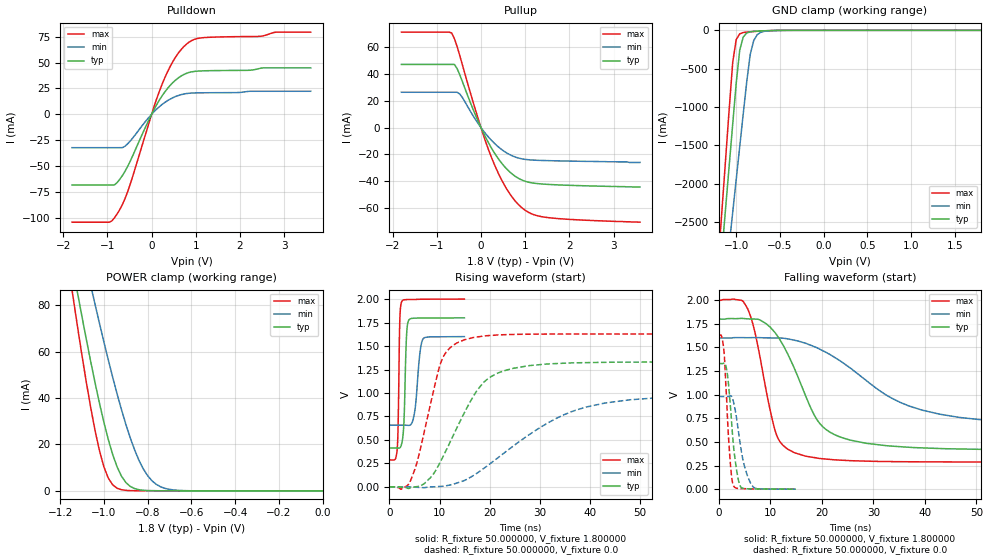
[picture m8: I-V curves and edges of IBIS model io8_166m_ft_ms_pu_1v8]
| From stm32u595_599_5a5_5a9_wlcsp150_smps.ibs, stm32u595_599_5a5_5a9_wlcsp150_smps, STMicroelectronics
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|   Model io8_166m_ft_ms_pu_1v8
[Model]  io8_166m_ft_ms_pu_1v8
Model_type I/O
Polarity   Non-Inverting
Enable   Active-Low
Vinl =   0.540000V
Vinh =   1.260000V
Vmeas =  0.900000V
Cref =   50.000000pF
Rref =   100.000000M
Vref =   0.0V
C_comp   3.358200pF   3.352700pF   3.400300pF
[Temperature Range]   25.000000   0.140000k   -40.000000
[Pullup Reference]   1.800000V   1.600000V   2.000000V
[Pulldown Reference]   0.0V   0.0V   0.0V
[POWER Clamp Reference]   1.800000V   1.600000V   2.000000V
[GND Clamp Reference]   0.0V   0.0V   0.0V
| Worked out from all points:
|   slope of the pulldown table from 0 to 0.27 V, typ, clamps not added: 13.6 ohm
|   slope of the pullup table from 0 to 0.27 V, typ, clamps not added: 15.9 ohm
|   GND clamp passes 1 mA (typ) near -0.51 V on its own axis
|   POWER clamp passes 1 mA (typ) near -0.86 V on its own axis
|   rising waveform, R_fixture 50.000000, V_fixture 1.800000: 20-80 % time 446ps typ, 896ps min, 294ps max; typ from 0.414 V to 1.8 V
|   rising waveform, R_fixture 50.000000, V_fixture 0.0: 20-80 % time 7.87ns typ, 16.8ns min, 4.3ns max; typ from 0 V to 1.33 V
|   falling waveform, R_fixture 50.000000, V_fixture 1.800000: 20-80 % time 7.17ns typ, 16.9ns min, 3.85ns max; typ from 1.8 V to 0.414 V
|   falling waveform, R_fixture 50.000000, V_fixture 0.0: 20-80 % time 1.31ns typ, 1.89ns min, 980ps max; typ from 1.33 V to 0 V
[Pulldown]
|Voltage   I(typ)   I(min)   I(max)
-1.8V     -68.38mA   -32.32mA   -104.4mA
-960mV    -68.38mA   -32.32mA   -104.4mA
-780mV    -66.08mA   -32.32mA   -96.43mA
-660mV    -59.2mA    -32.31mA   -87.22mA
-540mV    -50.22mA   -28.51mA   -74.66mA
0V        0A         0A         0A
240mV     18.04mA    9.6mA      29.42mA
480mV     30.68mA    16.02mA    50.95mA
780mV     39.48mA    19.99mA    67.56mA
1.14V     41.99mA    20.78mA    74.01mA
2.82V     44.92mA    22.27mA    79.53mA
3.6V      44.92mA    22.27mA    79.53mA
[Pullup]
|Voltage   I(typ)   I(min)   I(max)
-1.8V     47.02mA    26.28mA    71.09mA
-660mV    47.02mA    26.28mA    70.35mA
-600mV    47.02mA    26.28mA    66.17mA
-480mV    39.45mA    25.02mA    53.77mA
-60mV     4.42mA     2.808mA    6.308mA
240mV     -15.38mA   -9.6mA     -22.37mA
420mV     -24.43mA   -15.12mA   -35.87mA
600mV     -31.41mA   -19.24mA   -46.67mA
960mV     -39.54mA   -23.52mA   -60.64mA
1.2V      -41.44mA   -24.28mA   -64.93mA
1.56V     -42.42mA   -24.69mA   -67.24mA
3.6V      -44.3mA    -26mA      -70.5mA
[GND_clamp]
|Voltage   I(typ)   I(min)   I(max)
-1.8V     -9.908A    -9.683A    -9.994A
-1.2V     -3.383A    -4.084A    -2.934A
-1.16V    -2.841A    -3.655A    -2.294A
-1.12V    -2.299A    -3.226A    -1.656A
-1.04V    -1.218A    -2.369A    -414.2mA
-1V       -684.7mA   -1.941A    -119.2mA
-960mV    -257.2mA   -1.514A    -45.66mA
-920mV    -87.03mA   -1.089A    -28.93mA
-840mV    -19.35mA   -312.8mA   -18.97mA
-800mV    -13.55mA   -132.4mA   -15.49mA
-720mV    -8.042mA   -25.67mA   -9.491mA
1.8V      0A         13.64nA    0A
[POWER_clamp]
|Voltage   I(typ)   I(min)   I(max)
-1.8V     470.9mA    433.7mA    554.6mA
-1.14V    95.28mA    122.7mA    82.88mA
-1.12V    85mA       114mA      70.34mA
-1.06V    55.55mA    88.43mA    35.73mA
-1.04V    46.38mA    80.17mA    25.83mA
-1V       29.54mA    64.14mA    10.37mA
-940mV    10.43mA    41.88mA    1.177mA
-900mV    3.66mA     28.79mA    250.5uA
-840mV    527.2uA    13.26mA    95.95uA
-800mV    154uA      6.55mA     88.4uA
-740mV    59.84uA    1.741mA    70.38uA
0V        0A         18.18nA    0A
[Ramp]
| variable   typ   min   max
dV/dt_r  0.79757/7.86502n   0.58771/16.72662n   0.97651/4.29083n
dV/dt_f  0.83134/7.15391n   0.56288/16.90733n   1.02743/3.84506n
R_load = 50.000000
[Rising Waveform]
R_fixture= 50.000000
V_fixture= 1.800000
V_fixture_min= 1.600000
V_fixture_max= 2.000000
|time   V(typ)   V(min)   V(max)
0s        414.4mV    657.5mV    287.6mV
1.532ns   414mV      657.5mV    392.3mV
1.742ns   413.2mV    657.5mV    688.1mV
2.072ns   415.7mV    657.5mV    1.782V
2.432ns   457.2mV    657.5mV    1.971V
3.423ns   1.622V     656.4mV    1.995V
3.844ns   1.774V     655mV      1.995V
4.985ns   1.797V     782.4mV    1.996V
6.637ns   1.798V     1.57V      1.998V
14.95ns   1.8V       1.6V       2V
[Rising Waveform]
R_fixture= 50.000000
V_fixture= 0.0
V_fixture_min= 0.0
V_fixture_max= 0.0
|time   V(typ)   V(min)   V(max)
0s        427.6uV    510uV      389.4uV
4.204ns   -8.787mV   -259.1uV   66.17mV
7.007ns   38.17mV    -8.134mV   601mV
10.41ns   292.6mV    6.227mV    1.345V
15.02ns   796.5mV    70.05mV    1.568V
18.82ns   1.114V     196.9mV    1.606V
22.82ns   1.236V     358.6mV    1.62V
33.63ns   1.314V     738.7mV    1.627V
43.04ns   1.326V     893.4mV    1.628V
99.7ns    1.33V      980.7mV    1.628V
[Falling Waveform]
R_fixture= 50.000000
V_fixture= 1.800000
V_fixture_min= 1.600000
V_fixture_max= 2.000000
|time   V(typ)   V(min)   V(max)
0s        1.8V       1.6V       2V
5.606ns   1.803V     1.603V     1.91V
7.007ns   1.8V       1.604V     1.664V
11.01ns   1.651V     1.6V       606.8mV
14.81ns   1.26V      1.575V     383.9mV
20.22ns   659.2mV    1.465V     321.9mV
28.63ns   485.7mV    1.15V      297.1mV
36.84ns   444mV      882.4mV    290.4mV
46.85ns   425.7mV    758.5mV    288.4mV
99.7ns    414.4mV    657.5mV    287.6mV
[Falling Waveform]
R_fixture= 50.000000
V_fixture= 0.0
V_fixture_min= 0.0
V_fixture_max= 0.0
|time   V(typ)   V(min)   V(max)
0s        1.33V      980.7mV    1.628V
900.9ps   1.332V     980.7mV    1.517V
1.141ns   1.335V     980.7mV    1.366V
1.532ns   1.266V     980.5mV    954.2mV
2.252ns   885.8mV    987.8mV    276.9mV
2.883ns   449mV      919.1mV    34.91mV
4.114ns   40.19mV    499.6mV    6.396mV
4.985ns   6.659mV    244.8mV    5.402mV
6.366ns   3.244mV    46.7mV     3.649mV
14.95ns   427.6uV    510uV      389.4uV
